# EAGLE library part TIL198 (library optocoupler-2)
TEXAS INSTRUMENTS OPTO COUPLER
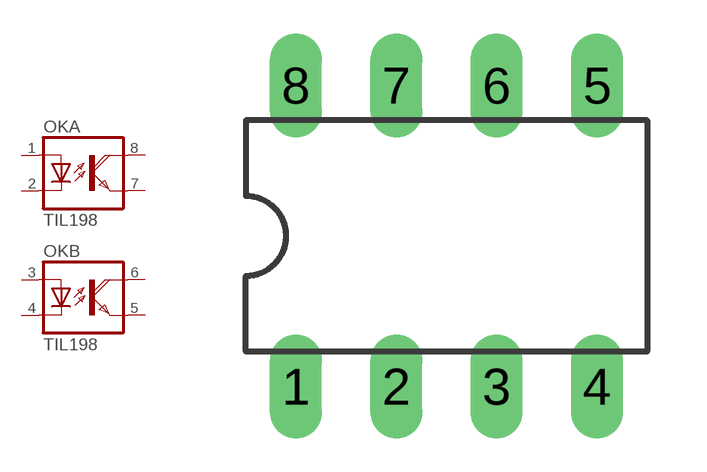
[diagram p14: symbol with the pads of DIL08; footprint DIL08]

Designator prefix OK; gates A=OK-D B=OK-D

## TIL198  [DIL08]
1  A:A  pas
2  A:C  pas
3  B:A  pas
4  B:C  pas
5  B:EMI  pas
6  B:COL  pas
7  A:EMI  pas
8  A:COL  pas

## Footprint DIL08 (pad centres in mm)
Dual In Line Package
drill 0.813 long: 1 -3.81,-3.81; 2 -1.27,-3.81; 3 1.27,-3.81; 4 3.81,-3.81; 5 3.81,3.81; 6 1.27,3.81; 7 -1.27,3.81; 8 -3.81,3.81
